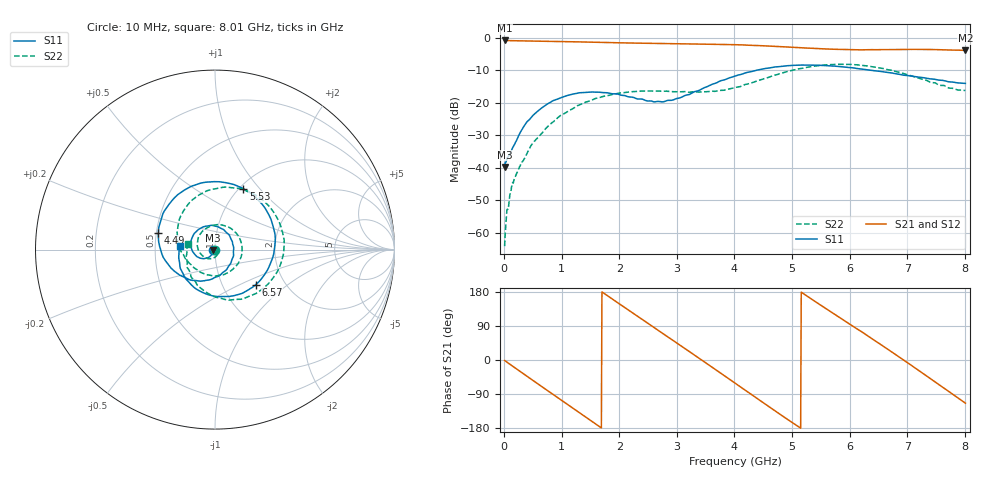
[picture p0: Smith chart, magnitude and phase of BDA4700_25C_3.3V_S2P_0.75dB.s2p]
!Agilent Technologies,E5071B,MY42404982,A.09.10
!Date: Mon Oct 20 18:03:17 2025
!Data & Calibration Information:
!Freq	S11:SOLT2(ON)	S21:SOLT2(ON)	S12:SOLT2(ON)	S22:SOLT2(ON)
# Hz S RI R 50
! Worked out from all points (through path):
!   801 points, 10 MHz to 8.01 GHz, reference 50 ohm
!   highest |S21| = -0.87 dB at 10 MHz (marker M1); lowest = -3.9 dB at 8.01 GHz (marker M2)
!   group delay of S21, straight-line fit = 288 ps
!   lowest |S11| = -39.7 dB at 10 MHz (marker M3), VSWR 1.02, Z = 49 - j0.226 ohm
!   |S11| at or under -10 dB: start of sweep to 4.39 GHz; 6.339 GHz to end of sweep
!   |S22| runs from -64.1 to -8.2 dB; largest |S21 - S12| = 0.01
!   S11 on the Smith chart (normalised r, x): 10 MHz: 0.98, -0.00; 4.49 GHz: 0.51, +0.11; 5.53 GHz: 1.04, +0.82; 6.57 GHz: 1.43, -0.62; 8.01 GHz: 0.67, +0.03
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1e7  -0.0101 -0.0023  0.9043 -0.0193  0.904 -0.0199  0.000212 -0.000589
1.5e8  -0.0133 -0.0155  0.86 -0.2528  0.8595 -0.2527  0.00354 0.0048
4.6e8  -0.0372 -0.0438  0.577 -0.6737  0.5767 -0.6739  0.0174 -0.0123
9e8  -0.1061 -0.0337  -0.0924 -0.8682  -0.092 -0.8686  -0.0227 -0.0508
1.35e9  -0.132 0.0537  -0.6899 -0.5099  -0.6902 -0.5102  -0.0955 0.00707
1.92e9  -0.0285 0.1341  -0.7678 0.3304  -0.7683 0.3305  -0.00764 0.136
2.32e9  0.0642 0.0941  -0.3505 0.7434  -0.3502 0.7434  0.1179 0.092
2.68e9  0.104 0.0118  0.1699 0.7955  0.1688 0.7948  0.1478 -0.0321
3.06e9  0.0776 -0.0905  0.6311 0.4991  0.6257 0.5036  0.0682 -0.1304
3.36e9  0.0095 -0.1512  0.7907 0.1016  0.7918 0.1017  -0.0217 -0.1437
3.67e9  -0.0979 -0.1734  0.7144 -0.3346  0.7144 -0.3366  -0.0998 -0.112
4.01e9  -0.2265 -0.1201  0.3775 -0.6804  0.3789 -0.679  -0.1618 -0.0537
4.49e9  -0.3157 0.0952  -0.2757 -0.6964  -0.2756 -0.6987  -0.2109 0.0941
4.92e9  -0.2026 0.3097  -0.6582 -0.2861  -0.6567 -0.2899  -0.1317 0.2722
5.35e9  0.0494 0.3748  -0.642 0.2388  -0.6435 0.2353  0.1024 0.3437
5.53e9  0.158 0.3385  -0.5271 0.4186  -0.5282 0.4174  0.213 0.3102
6.05e9  0.3349 0.0781  0.00225 0.6505  0.000234 0.6542  0.3848 0.0331
6.57e9  0.2265 -0.1958  0.5174 0.4007  0.518 0.3988  0.2361 -0.2397
6.68e9  0.1747 -0.2314  0.5853 0.2922  0.5867 0.2913  0.1795 -0.2644
7.23e9  -0.0892 -0.2287  0.5657 -0.338  0.5659 -0.3388  -0.0683 -0.2229
7.62e9  -0.1913 -0.1085  0.1964 -0.6192  0.1968 -0.6194  -0.1542 -0.1013
8.01e9  -0.1969 0.0208  -0.258 -0.5818  -0.2559 -0.5833  -0.1508 0.0302
